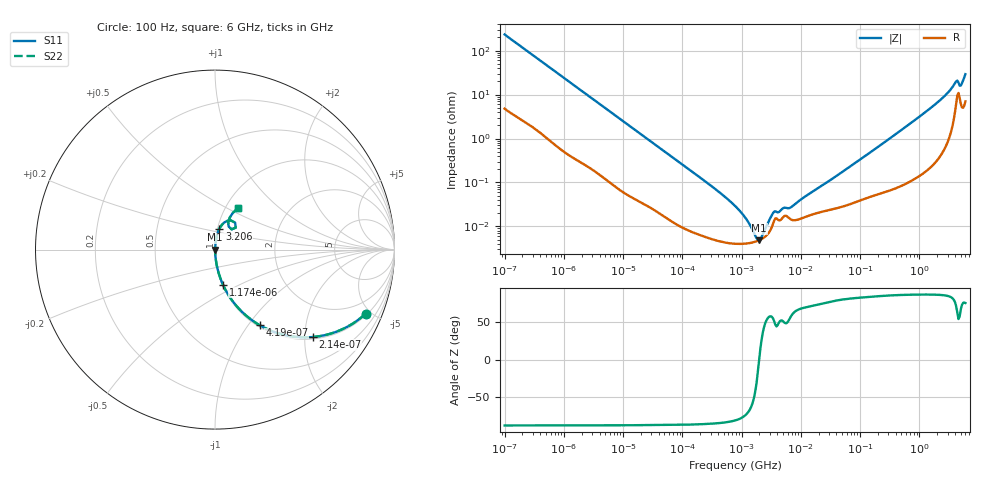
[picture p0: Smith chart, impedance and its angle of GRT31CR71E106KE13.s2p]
!Murata Part Number: GRT31CR71E106KE13
!These Parameters are Measured in Series Mode Connection
!Data Generated on Jun 19, 2026
!  o--ll--o
!Port1  Port2
!  o------o
!Operation Temp=25[degC], DC Bias Voltage=0[V]
!Freq. Start=100[Hz] Stop=6[GHz] 401[Steps]
# Hz S RI R 50
!Freq.(Hz) S11(Real) S11(Imag) S21(Real) S21(Imag) S12(Real) S12(Imag) S22(Real) S22(Imag)
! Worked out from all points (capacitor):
!   401 points, 100 Hz to 6 GHz, reference 50 ohm
!   read as one part in series: C = 6.8 uF near 109 Hz
!   lowest |Z| = 4.86 mohm at 1.983 MHz (marker M1)
!   S11 on the Smith chart (normalised r, x): 100 Hz: 1.10, -4.66; 214 Hz: 1.05, -2.20; 419 Hz: 1.03, -1.13; 1.174 kHz: 1.01, -0.41; 3.206 GHz: 1.02, +0.24; 6 GHz: 1.14, +0.56
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100  0.8395 -0.357  0.1605 0.357  0.1605 0.357  0.8395 -0.357
214  0.546 -0.4869  0.454 0.4869  0.454 0.4869  0.546 -0.4869
419  0.2486 -0.421  0.7514 0.421  0.7514 0.421  0.2486 -0.421
686  0.1138 -0.3072  0.8862 0.3072  0.8862 0.3072  0.1138 -0.3072
1174  0.0442 -0.1953  0.9558 0.1953  0.9558 0.1953  0.0442 -0.1953
2008  0.017 -0.1184  0.983 0.1184  0.983 0.1184  0.017 -0.1184
6433  0.00239 -0.0383  0.9976 0.0383  0.9976 0.0383  0.00239 -0.0383
40335  0.000241 -0.0063  0.9998 0.0063  0.9998 0.0063  0.000241 -0.0063
330837  5.1e-05 -0.000773  0.9999 0.000773  0.9999 0.000773  5.1e-05 -0.000773
774597  4.04e-05 -0.000291  1 0.000291  1 0.000291  4.04e-05 -0.000291
1449809  4.25e-05 -8.66e-05  1 8.66e-05  1 8.66e-05  4.25e-05 -8.66e-05
1983483  4.86e-05 0  1 0  1 0  4.86e-05 0
2594782  6.13e-05 7.78e-05  0.9999 -7.78e-05  0.9999 -7.78e-05  6.13e-05 7.78e-05
3549919  0.000135 0.00017  0.9999 -0.00017  0.9999 -0.00017  0.000135 0.00017
6948629  0.000142 0.000238  0.9999 -0.000238  0.9999 -0.000238  0.000142 0.000238
1.555665e7  0.000187 0.000582  0.9998 -0.000582  0.9998 -0.000582  0.000187 0.000582
3.124326e8  0.000749 0.00986  0.9993 -0.00986  0.9993 -0.00986  0.000749 0.00986
1.565993e9  0.00469 0.0495  0.9953 -0.0495  0.9953 -0.0495  0.00469 0.0495
3.205649e9  0.024 0.1153  0.976 -0.1153  0.976 -0.1153  0.024 0.1153
4.009986e9  0.0662 0.1592  0.9338 -0.1592  0.9338 -0.1592  0.0662 0.1592
5.016141e9  0.0761 0.1285  0.9239 -0.1285  0.9239 -0.1285  0.0761 0.1285
6e9  0.1264 0.2306  0.8736 -0.2306  0.8736 -0.2306  0.1264 0.2306
